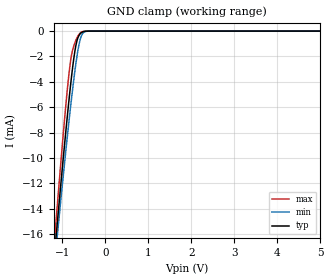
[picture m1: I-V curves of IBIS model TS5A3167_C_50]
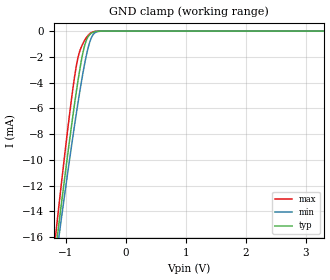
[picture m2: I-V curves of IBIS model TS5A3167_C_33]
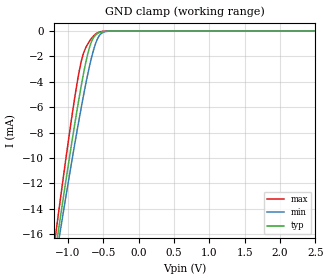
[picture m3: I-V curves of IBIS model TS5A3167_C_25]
| TEXAS INSTRUMENTS INCORPORATED
| Standard Linear and Logic Group
| IBIS Model of TS5A3167
| 1-OHM SPST ANALOG SWITCH
| This file contains package information for the following:
|  SOT 5-pin (DCK) package as [Component] TS5A3167_DCK
|  SOT 5-pin (DBV) package as [Component] TS5A3167_DBV
| This device can be powered at the following Vccs:
|  5 volt Vcc
|  3.3 volt Vcc
|  2.5 volt Vcc
|  1.8 volt Vcc
| This file provides unique models under the [Model Selector] for each Vcc.
| For operation at a specific Vcc, select the appropriate model after each
| [Model Selector] keyword.
[IBIS Ver]   3.2
[Comment char]  |_char
[File Name]   ts5a3167.ibs
[File Rev]   1.1 | a_die
[Date]   January 25, 2005
[Source]   Data created from TI-SPICE simulations at TI-SLL.
[Notes]   The following is an IBIS list for the TS5A3167.
   Please contact sllibis@ti.com with questions and
   comments concerning SLL IBIS models.
   - FILE REV HISTORY
   - 1.1 Release IBIS file on 01/31/05
   - Power clamp data deleted in the IN models as there
   is no power-clamp diode.
   - Non-monotonic data due to FET characteristics.
   - NCH & PCH MOSFETS, so [Series Mosfet] model can have rising
   or falling currents
[Disclaimer] Property of Texas Instruments Incorporated.  Unauthorized
   reproduction and/or distribution is strictly prohibited.
   This product is protected under copyright law.
   Created  2005, (C) Copyright  2005, Texas Instruments
   Incorporated, All Rights Reserved
   UNLESS THERE IS A SIGNED, WRITTEN AGREEMENT TO THE
   CONTRARY, TEXAS INSTRUMENTS (TI) IS PROVIDING THE IBIS
   MODELS  AND WITHOUT ANY WARRANTY, EXPRESSED OR
   IMPLIED.  TI assumes no liability for:
   1) the accuracy of the IBIS models provided to your
   company;
   2) the proper functioning of these IBIS Models in your
   design or for any resulting applications; or
   3) infringement of patents, copyrights or intellectual
   property rights resulting from your use of these IBIS
   models.
   TI provides IBIS Models as a service to our customers.
   You and your company shall not distribute, sell or give
   these models to anyone else without prior written
   permission from TI.
   TI reserves the right to make changes to our products or
   to discontinue any semiconductor product or service
   without notice, and advises our customers to obtain the
   latest version of relevant information to verify, before
   placing orders, that the information being relied on is
   current.
   Please be aware that your receipt and use of the IBIS
   information provided shall serve as acceptance of these
   terms and conditions.  If you do not accept these terms,
   you should return or destroy the IBIS models and any
   other accompanying information immediately.
| Component TS5A3167_DCK 5-pin SOT
[Component]   TS5A3167_DCK
[Manufacturer]   Texas Instruments, Inc.
[Package]
|   typ   min   max
R_pkg   2.000e-02   1.700e-02   2.500e-02
L_pkg   9.980e-10   8.810e-10   1.069e-09
C_pkg   1.460e-13   1.180e-13   2.050e-13
[Pin]   signal_name   model_name   R_pin   L_pin   C_pin
1   NC   TS5A3167_A   1.900e-02   1.069e-09   1.620e-13
2   COM   TS5A3167_B   1.800e-02   8.810e-10   1.210e-13
3   GND   GND   1.700e-02   1.031e-09   2.050e-13
4   IN   TS5A3167_C   2.000e-02   9.600e-10   1.240e-13
5   VCC   POWER   2.500e-02   1.049e-09   1.180e-13
| Component TS5A3167_DBV 5-pin SOT
[Component]   TS5A3167_DBV
[Manufacturer]   Texas Instruments, Inc.
[Package]
|   typ   min   max
R_pkg   2.500e-02   2.100e-02   2.900e-02
L_pkg   1.529e-09   1.312e-09   1.906e-09
C_pkg   1.560e-13   1.100e-13   2.400e-13
[Pin]   signal_name   model_name   R_pin   L_pin   C_pin
1   NO   TS5A3167_A   2.100e-02   1.511e-09   1.440e-13
2   COM   TS5A3167_B   2.300e-02   1.312e-09   1.380e-13
3   GND   GND   2.900e-02   1.906e-09   2.400e-13
4   IN   TS5A3167_C   2.600e-02   1.541e-09   1.500e-13
5   VCC   POWER   2.500e-02   1.374e-09   1.100e-13
[Series Switch Groups]
| Function Group States
On  1 /   | A->B C LOW
On  2 /   | B->A C LOW
Off 1 2 /   | C HIGH
[Series Pin Mapping]   pin_2   model_name   function_table_group
1   2   TS5A3167_A_50_S   1
| 1   2   TS5A3167_A_33_S   1
| 1   2   TS5A3167_A_25_S   1
| 1   2   TS5A3167_A_18_S   1
2   1   TS5A3167_B_50_S   2
| 2   1   TS5A3167_B_33_S   2
| 2   1   TS5A3167_B_25_S   2
| 2   1   TS5A3167_B_18_S   2
| Model TS5A3167_C
[Model Selector]   TS5A3167_C
TS5A3167_C_50   5 volt Vcc
TS5A3167_C_33   3.3 volt Vcc
TS5A3167_C_25   2.5 volt Vcc
TS5A3167_C_18   1.8 volt Vcc
| Model TS5A3167_A
[Model Selector]   TS5A3167_A
TS5A3167_A_50   5 volt Vcc
TS5A3167_A_33   3.3 volt Vcc
TS5A3167_A_25   2.5 volt Vcc
TS5A3167_A_18   1.8 volt Vcc
| Model TS5A3167_A_S
[Model Selector]   TS5A3167_A_S
TS5A3167_A_50_S   5 volt Vcc_S
TS5A3167_A_33_S   3.3 volt Vcc_S
TS5A3167_A_25_S   2.5 volt Vcc_S
TS5A3167_A_18_S   1.8 volt Vcc_S
| Model TS5A3167_B
[Model Selector]   TS5A3167_B
TS5A3167_B_50   5 volt Vcc
TS5A3167_B_33   3.3 volt Vcc
TS5A3167_B_25   2.5 volt Vcc
TS5A3167_B_18   1.8 volt Vcc
| Model TS5A3167_B_S
[Model Selector]   TS5A3167_B_S
TS5A3167_B_50_S   5 volt Vcc_S
TS5A3167_B_33_S   3.3 volt Vcc_S
TS5A3167_B_25_S   2.5 volt Vcc_S
TS5A3167_B_18_S   1.8 volt Vcc_S
[Model]   TS5A3167_A_50_S
Model_type  Series_switch
| variable   typ   min   max
C_comp   0   0   0
[Temperature Range]   40   100   -40
| Ambient temperature   25   85   -40
[Voltage range]   5   4.5   5.5
[On]
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[Off]
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[Model]   TS5A3167_A_33_S
Model_type  Series_switch
| variable   typ   min   max
C_comp   0   0   0
[Temperature Range]   40   100   -40
| Ambient temperature   25   85   -40
[Voltage range]   3.3   3   3.6
[On]
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[Off]
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[Model]   TS5A3167_A_25_S
Model_type  Series_switch
| variable   typ   min   max
C_comp   0   0   0
[Temperature Range]   40   100   -40
| Ambient temperature   25   85   -40
[Voltage range]   2.5   2.3   2.7
[On]
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[Off]
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[Model]   TS5A3167_A_18_S
Model_type  Series_switch
| variable   typ   min   max
C_comp   0   0   0
[Temperature Range]   40   100   -40
| Ambient temperature   25   85   -40
[Voltage range]   1.8   1.65   1.95
[On]
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[Off]
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[Model]   TS5A3167_B_50_S
Model_type  Series_switch
| variable   typ   min   max
C_comp   0   0   0
[Temperature Range]   40   100   -40
| Ambient temperature   25   85   -40
[Voltage range]   5   4.5   5.5
[On]
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[Off]
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[Model]   TS5A3167_B_33_S
Model_type  Series_switch
| variable   typ   min   max
C_comp   0   0   0
[Temperature Range]   40   100   -40
| Ambient temperature   25   85   -40
[Voltage range]   3.3   3   3.6
[On]
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[Off]
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[Model]   TS5A3167_B_25_S
Model_type  Series_switch
| variable   typ   min   max
C_comp   0   0   0
[Temperature Range]   40   100   -40
| Ambient temperature   25   85   -40
[Voltage range]   2.5   2.3   2.7
[On]
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[Off]
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[Model]   TS5A3167_B_18_S
Model_type  Series_switch
| variable   typ   min   max
C_comp   0   0   0
[Temperature Range]   40   100   -40
| Ambient temperature   25   85   -40
[Voltage range]   1.8   1.65   1.95
[On]
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[Off]
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| Models and submodels in the file (20): TS5A3167_C_50 (Input), TS5A3167_C_33 (Input), TS5A3167_C_25 (Input), TS5A3167_C_18 (Input), TS5A3167_A_50_S (Series_switch), TS5A3167_A_50 (Terminator), TS5A3167_A_33_S (Series_switch), TS5A3167_A_33 (Terminator), TS5A3167_A_25_S (Series_switch), TS5A3167_A_25 (Terminator), TS5A3167_A_18_S (Series_switch), TS5A3167_A_18 (Terminator), TS5A3167_B_50_S (Series_switch), TS5A3167_B_50 (Terminator), TS5A3167_B_33_S (Series_switch), TS5A3167_B_33 (Terminator), TS5A3167_B_25_S (Series_switch), TS5A3167_B_25 (Terminator), TS5A3167_B_18_S (Series_switch), TS5A3167_B_18 (Terminator)
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[Model]   TS5A3167_C_50
Model_type  Input
Vinl=0.8
Vinh=2.4
| variable   typ   min   max
C_comp   1.62pF   1.26pF   2.18pF
[Temperature Range]   40   100   -40
| Ambient temperature   25   85   -40
[Voltage range]   5   4.5   5.5
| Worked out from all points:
|   GND clamp passes 1 mA (typ) near -0.68 V on its own axis
[GND Clamp]
| TS5A3167_C_50
|   Voltage   I(typ)   I(min)   I(max)
-5V       -179mA     -167.3mA   -192.5mA
-1.19V    -17.81mA   -18.6mA    -16.71mA
-1.155V   -16.48mA   -17.37mA   -15.23mA
-1.12V    -15.16mA   -16.15mA   -13.77mA
-1.085V   -13.84mA   -14.95mA   -12.32mA
-930mV    -8.226mA   -9.739mA   -6.188mA
-820mV    -4.56mA    -6.261mA   -2.59mA
-770mV    -3.071mA   -4.78mA    -1.597mA
-685mV    -1.109mA   -2.515mA   -710.1uA
-610mV    -317.2uA   -994.2uA   -241.2uA
-545mV    -93.94uA   -277.4uA   -57.32uA
5V        84.64pA    185.3pA    50.23pA
[Model]   TS5A3167_C_33
Model_type  Input
Vinl=0.8
Vinh=2.0
| variable   typ   min   max
C_comp   1.67pF   1.33pF   2.13pF
[Temperature Range]   40   100   -40
| Ambient temperature   25   85   -40
[Voltage range]   3.3   3   3.6
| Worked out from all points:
|   GND clamp passes 1 mA (typ) near -0.68 V on its own axis
[GND Clamp]
| TS5A3167_C_33
|   Voltage   I(typ)   I(min)   I(max)
-3.3V     -105.4mA   -99.17mA   -112.8mA
-1.165V   -16.86mA   -17.72mA   -15.65mA
-1.14V    -15.91mA   -16.85mA   -14.6mA
-1.11V    -14.78mA   -15.81mA   -13.35mA
-1.085V   -13.84mA   -14.95mA   -12.32mA
-920mV    -7.878mA   -9.413mA   -5.819mA
-820mV    -4.56mA    -6.261mA   -2.59mA
-765mV    -2.933mA   -4.637mA   -1.526mA
-690mV    -1.195mA   -2.636mA   -750.5uA
-570mV    -153.7uA   -480.2uA   -105.7uA
-375mV    -1.347uA   -3.104uA   -200.4nA
3.3V      52.93pA    130.9pA    33.09pA
[Model]   TS5A3167_C_25
Model_type  Input
Vinl=0.6
Vinh=1.8
| variable   typ   min   max
C_comp   1.71pF   1.38pF   2.09pF
[Temperature Range]   40   100   -40
| Ambient temperature   25   85   -40
[Voltage range]   2.5   2.3   2.7
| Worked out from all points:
|   GND clamp passes 1 mA (typ) near -0.68 V on its own axis
[GND Clamp]
| TS5A3167_C_25
|   Voltage   I(typ)   I(min)   I(max)
-2.5V     -71.31mA   -67.74mA   -75.63mA
-1.17V    -17.05mA   -17.9mA    -15.87mA
-1.145V   -16.1mA    -17.02mA   -14.81mA
-1.1V     -14.4mA    -15.46mA   -12.94mA
-925mV    -8.052mA   -9.576mA   -6.003mA
-825mV    -4.716mA   -6.413mA   -2.719mA
-770mV    -3.071mA   -4.78mA    -1.597mA
-700mV    -1.38mA    -2.884mA   -834.7uA
-590mV    -222.5uA   -707.5uA   -163.6uA
-520mV    -55.2uA    -151.1uA   -29.07uA
-425mV    -5.375uA   -12.08uA   -1.336uA
2.5V      39.8pA     107.9pA    25.06pA
